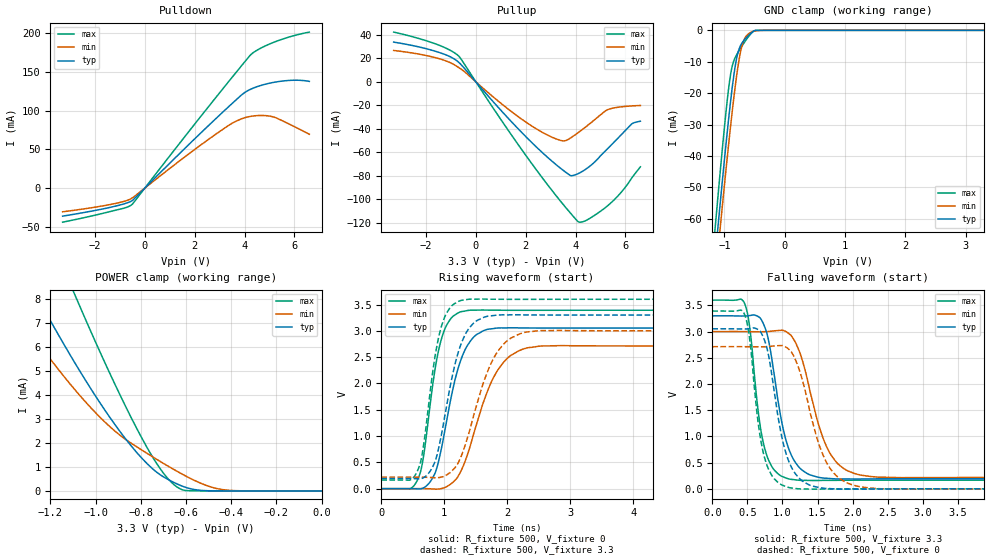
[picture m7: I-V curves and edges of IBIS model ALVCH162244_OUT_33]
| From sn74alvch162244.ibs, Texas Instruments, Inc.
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[Model]   ALVCH162244_OUT_33
Model_type  3-state
Enable   Active-Low
Vref =   0
Rref =   500
Cref =   50p
Vmeas =   1.5
| variable   typ   min   max
C_comp   6.78pF   5.69pF   8.02pF
| C_pullup   4.88pF   3.79pF   7.05pF
| C_pulldown   4.24pF   3.61pF   5.42pF
| C_tri-state   6.78pF   5.69pF   8.02pF
[Temperature Range]   40   100   -40
| Ambient temperature   25   85   -40
[Voltage range]   3.3   3   3.6
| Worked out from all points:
|   slope of the pulldown table from 0 to 0.495 V, typ, clamps not added: 31 ohm
|   slope of the pullup table from 0 to 0.495 V, typ, clamps not added: 40.8 ohm
|   GND clamp passes 1 mA (typ) near -0.57 V on its own axis
|   POWER clamp passes 1 mA (typ) near -0.76 V on its own axis
|   rising waveform, R_fixture 500, V_fixture 0: 20-80 % time 336ps typ, 471ps min, 247ps max; typ from 0 V to 3.05 V
|   falling waveform, R_fixture 500, V_fixture 3.3: 20-80 % time 253ps typ, 355ps min, 183ps max; typ from 3.3 V to 0.192 V
|   rising waveform, R_fixture 500, V_fixture 3.3: 20-80 % time 327ps typ, 452ps min, 243ps max; typ from 0.193 V to 3.3 V
|   falling waveform, R_fixture 500, V_fixture 0: 20-80 % time 250ps typ, 350ps min, 184ps max; typ from 3.05 V to 0 V
[GND Clamp]
| ALVCH162244_OUT_33
|   Voltage   I(typ)   I(min)   I(max)
-3.3V     -548.4mA   -542.7mA   -558.5mA
-1.155V   -72.51mA   -79.89mA   -63.21mA
-1.115V   -64.26mA   -71.86mA   -54.58mA
-1.075V   -56.11mA   -63.91mA   -46.11mA
-1.06V    -53.1mA    -60.96mA   -42.98mA
-920mV    -26.42mA   -34.46mA   -16.98mA
-870mV    -18.13mA   -25.74mA   -11.35mA
-810mV    -10.18mA   -16.26mA   -8.23mA
-750mV    -5.602mA   -8.606mA   -6.242mA
-695mV    -3.671mA   -4.077mA   -4.581mA
-555mV    -813.6uA   -545.2uA   -989uA
3.3V      114.4pA    971.2nA    51.31pA
[POWER Clamp]
| ALVCH162244_OUT_33
|   Voltage   I(typ)   I(min)   I(max)
-3.3V     50.81mA    40.09mA    67.1mA
-1.4V     10.61mA    8.137mA    15.34mA
-1.26V    8.125mA    6.259mA    12.01mA
-1.085V   5.24mA     4.151mA    8.039mA
-940mV    3.112mA    2.71mA     4.968mA
-815mV    1.573mA    1.823mA    2.555mA
-715mV    679.8uA    1.235mA    940uA
-645mV    315uA      848.1uA    201uA
-600mV    145.4uA    616.5uA    16.03uA
-505mV    8.927uA    212.2uA    391.2nA
-435mV    705.2nA    51.1uA     24.12nA
-48.03fV  114.4pA    365.2pA    62.68pA
[Pulldown]
| ALVCH162244_OUT_33
|   Voltage   I(typ)   I(min)   I(max)
-3.3V     -36.3mA    -30.69mA   -44.1mA
-1.34V    -24.58mA   -20.97mA   -29.91mA
-765mV    -19.72mA   -16.5mA    -25.27mA
-515mV    -16.42mA   -12.96mA   -21.23mA
2.61V     82.41mA    64.15mA    107.4mA
3.46V     108mA      82.94mA    141.4mA
3.98V     122.8mA    90.59mA    162mA
4.365V    129.3mA    93.17mA    175.3mA
4.765V    133.6mA    93.71mA    182.6mA
5.12V     136.2mA    92.18mA    187.6mA
5.925V    139.3mA    80.56mA    196.4mA
6.6V      137.8mA    69.48mA    201.5mA
[Pullup]
| ALVCH162244_OUT_33
|   Voltage   I(typ)   I(min)   I(max)
-3.3V     33.84mA    26.74mA    42.38mA
-1.565V   25.66mA    20.28mA    31.92mA
-685mV    16.58mA    12.1mA     21.83mA
1.37V     -32.66mA   -24.4mA    -43.47mA
2.71V     -61.07mA   -43.5mA    -82.96mA
3.535V    -75.83mA   -50.28mA   -105.2mA
3.815V    -79.87mA   -47.52mA   -112.3mA
4.11V     -78.06mA   -43.16mA   -119.1mA
4.475V    -73.37mA   -37.22mA   -117.4mA
5.285V    -56.89mA   -23.71mA   -105.5mA
6.245V    -35.97mA   -20.5mA    -82.12mA
6.6V      -33.5mA    -20.1mA    -72.33mA
[Ramp]
| ALVCH162244_OUT_33
| variable   typ   min   max
dV/dt_r   1.84/3.38E-10   1.64/4.86E-10   2.04/2.55E-10
dV/dt_f   1.88/2.65E-10   1.69/3.74E-10   2.08/1.88E-10
R_load = 500
[Rising Waveform]
| ALVCH162244_OUT_33
R_fixture =   500
C_fixture =   0
L_fixture =   0
V_fixture =   0
V_fixture_min = 0
V_fixture_max = 0
|   Time   V(typ)   V(min)   V(max)
0s        276.4uV    305.8uV    244uV
565ps     -3.099mV   2.503mV    144mV
665ps     12.67mV    1.9mV      575.5mV
805ps     184.6mV    -4.525mV   1.874V
1.025ns   1.21V      31.02mV    3.079V
1.215ns   2.268V     226.2mV    3.338V
1.415ns   2.806V     824.9mV    3.393V
1.88ns    3.056V     2.307V     3.392V
2.575ns   3.053V     2.715V     3.391V
40ns      3.053V     2.712V     3.391V
[Falling Waveform]
| ALVCH162244_OUT_33
R_fixture =   500
C_fixture =   0
L_fixture =   0
V_fixture =   3.3
V_fixture_min = 3
V_fixture_max = 3.6
|   Time   V(typ)   V(min)   V(max)
0s        3.3V       3V         3.6V
465ps     3.297V     2.999V     3.518V
540ps     3.307V     2.998V     3.004V
700ps     3.222V     2.996V     1.054V
805ps     2.805V     3.002V     536.5mV
1.035ns   1.002V     3.009V     213.4mV
1.245ns   398.5mV    2.607V     162.5mV
1.69ns    194.5mV    650.6mV    161.1mV
2.365ns   189.6mV    222.3mV    164.6mV
40ns      192.3mV    217.1mV    164.5mV
[Rising Waveform]
| ALVCH162244_OUT_33
R_fixture =   500
C_fixture =   0
L_fixture =   0
V_fixture =   3.3
V_fixture_min = 3
V_fixture_max = 3.6
|   Time   V(typ)   V(min)   V(max)
0s        192.6mV    217.4mV    164.8mV
560ps     188.7mV    219.3mV    303mV
655ps     200.1mV    218.6mV    700.3mV
790ps     360.2mV    212.4mV    1.975V
1.015ns   1.428V     246.5mV    3.286V
1.205ns   2.523V     454.9mV    3.548V
1.405ns   3.065V     1.115V     3.602V
1.855ns   3.301V     2.619V     3.6V
2.535ns   3.302V     3.005V     3.599V
40ns      3.3V       3V         3.6V
[Falling Waveform]
| ALVCH162244_OUT_33
R_fixture =   500
C_fixture =   0
L_fixture =   0
V_fixture =   0
V_fixture_min = 0
V_fixture_max = 0
|   Time   V(typ)   V(min)   V(max)
0s        3.052V     2.711V     3.391V
465ps     3.05V      2.711V     3.305V
530ps     3.057V     2.71V      2.872V
695ps     2.978V     2.709V     890.1mV
800ps     2.554V     2.714V     377.1mV
1.025ns   793.1mV    2.721V     55.72mV
1.25ns    185.2mV    2.226V     -2.385mV
1.675ns   3.96mV     396.9mV    -4.246mV
2.385ns   -3.08mV    1.462mV    -52.39uV
40ns      544.7pV    6.131nV    695.6pV
